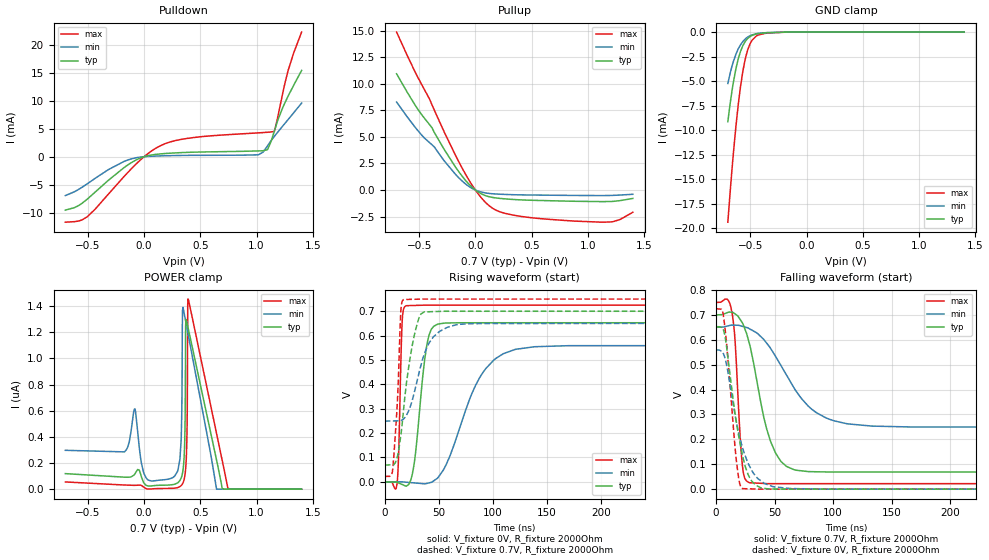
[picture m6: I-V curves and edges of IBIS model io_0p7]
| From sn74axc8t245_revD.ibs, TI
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|   io_0p7 Model
[Model]   io_0p7
Model_type   I/O
Polarity   Non-Inverting
Enable   Active-High
Vinl = 0.21
Vinh = 0.49
Vmeas = 0.35
Vref = 0
Cref = 2pF
Rref = 100000
|   typ   min   max
C_comp   1.54049E-12   1.37923E-12   1.78504E-12
[Model spec]
|subparameter
Vinl   0.21   0.195   0.225
Vinh   0.49   0.455   0.525
| Where Nom  PVT is Nominal Process, 0.7V, 27C
|   Fast PVT is Strong Process,  0.75V, -40C
|   Slow PVT is Weak Process,   0.65, 130C
[Voltage Range]   0.7   0.65   0.75
|Junction Temperature
[Temperature Range]   27   130   -40
[Pullup Reference]   0.7   0.65   0.75
[Pulldown Reference]   0   0   0
[Power Clamp Reference]   0.7   0.65   0.75
[GND Clamp Reference]   0   0   0
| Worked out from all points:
|   slope of the pulldown table from 0 to 0.105 V, typ, clamps not added: 251 ohm
|   slope of the pullup table from 0 to 0.105 V, typ, clamps not added: 180 ohm
|   GND clamp passes 1 mA (typ) near -0.55 V on its own axis
|   falling waveform, V_fixture 0.7V, R_fixture 2000Ohm: 20-80 % time 17.3ns typ, 33.8ns min, 5.11ns max; typ from 0.7 V to 0.069 V
|   rising waveform, V_fixture 0V, R_fixture 2000Ohm: 20-80 % time 8.82ns typ, 29.9ns min, 2.41ns max; typ from 0 V to 0.653 V
|   rising waveform, V_fixture 0.7V, R_fixture 2000Ohm: 20-80 % time 11ns typ, 16ns min, 4.59ns max; typ from 0.069 V to 0.7 V
|   falling waveform, V_fixture 0V, R_fixture 2000Ohm: 20-80 % time 12.5ns typ, 15.7ns min, 7.58ns max; typ from 0.653 V to 0 V
[Pulldown]
|   Voltage   I(typ)   I(min)   I(max)
-700mV    -9.53mA    -6.936mA   -11.68mA
-504.7mV  -7.56mA    -4.826mA   -10.71mA
-116.2mV  -1.094mA   -401.5uA   -2.212mA
-700uV    -4.135uA   -1.175uA   -12.02uA
156.8mV   524.2uA    153.9uA    2.074mA
444.5mV   814.4uA    247.4uA    3.433mA
1.016V    1.034mA    340.2uA    4.259mA
1.058V    1.067mA    839.6uA    4.313mA
1.098V    1.317mA    1.959mA    4.368mA
1.156V    4.475mA    3.596mA    4.506mA
1.278V    10.74mA    6.591mA    15.25mA
1.4V      15.4mA     9.579mA    22.24mA
[GND Clamp]
|   Voltage   I(typ)   I(min)   I(max)
-700mV    -9.134mA   -5.242mA   -19.38mA
-664.3mV  -6.083mA   -3.529mA   -14.17mA
-630.7mV  -3.882mA   -2.333mA   -9.91mA
-605.5mV  -2.655mA   -1.67mA    -7.215mA
-567.7mV  -1.415mA   -980.1uA   -4.082mA
-544.6mV  -944.1uA   -698.3uA   -2.722mA
-521.5mV  -629.7uA   -495uA     -1.75mA
-483.7mV  -335.9uA   -282.4uA   -814.3uA
-445.9mV  -193.6uA   -164.6uA   -387.5uA
-351.4mV  -64.76uA   -49.97uA   -92.43uA
-175mV    -4.252uA   -4.028uA   -4.183uA
1.4V      0A         0A         0A
[Pullup]
|   Voltage   I(typ)   I(min)   I(max)
-700mV    10.94mA    8.279mA    14.86mA
-511mV    7.597mA    5.59mA     10.6mA
-385mV    5.85mA     4.251mA    8.008mA
-275.8mV  3.798mA    2.733mA    5.441mA
-116.2mV  1.282mA    830.6uA    2.039mA
-700uV    5.462uA    3.045uA    10.64uA
129.5mV   -653.1uA   -334uA     -1.541mA
213.5mV   -787.5uA   -396.1uA   -2.037mA
360.5mV   -908.5uA   -451.5uA   -2.409mA
881.3mV   -1.064mA   -514.5uA   -2.93mA
1.222V    -1.075mA   -509.2uA   -2.989mA
1.4V      -796uA     -406uA     -2.097mA
[POWER Clamp]
|   Voltage   I(typ)   I(min)   I(max)
-700mV    118.8nA    297.2nA    55.28nA
-82.6mV   116.1nA    614.3nA    29.33nA
18.2mV    29.94nA    86.4nA     4.018nA
255.5mV   34.86nA    88.97nA    6.633nA
318.5mV   66.18nA    231.3nA    19.67nA
337.4mV   106.9nA    801.1nA    35.29nA
341.6mV   123.5nA    1.369uA    41.03nA
360.5mV   347.9nA    1.325uA    93.15nA
379.4mV   1.28uA     1.24uA     350.7nA
389.9mV   1.239uA    1.192uA    1.454uA
744.8mV   0A         0A         6.021nA
1.4V      0A         0A         0A
[Ramp]
R_load = 2000
|   typ   min   max
dV/dt_r   0.391697/8.77565e-09   0.335547/2.98927e-08   0.434999/2.39639e-09
dV/dt_f   0.378832/1.72731e-08   0.240634/3.38318e-08   0.436699/5.08929e-09
[Falling Waveform]
V_fixture = 0.7V
V_fixture_min = 0.65V
V_fixture_max = 0.75V
R_fixture = 2000Ohm
C_fixture = 0F
|   Time   V(typ)   V(min)   V(max)
0s        700mV      650mV      750mV
13.57ns   710.5mV    659mV      711mV
16.42ns   703.2mV    658.6mV    584.9mV
22.45ns   668.6mV    654.1mV    98.27mV
28.31ns   587.6mV    644.9mV    26.3mV
46.67ns   191mV      564.7mV    22.2mV
67.52ns   77.03mV    399.7mV    22.2mV
93.66ns   69.19mV    286.8mV    22.2mV
133.2ns   68.71mV    253.3mV    22.19mV
500ns     68.61mV    248.9mV    22.17mV
[Rising Waveform]
V_fixture = 0V
V_fixture_min = 0V
V_fixture_max = 0V
R_fixture = 2000Ohm
C_fixture = 0F
|   Time   V(typ)   V(min)   V(max)
0s        923.3nV    12.36uV    39.3nV
11.32ns   -1.698mV   -323.5uV   -9.278mV
16.05ns   -11mV      -463.7uV   653.2mV
19.76ns   -18.13mV   -1.707mV   722.7mV
27.05ns   70.28mV    -4.537mV   723.7mV
39.15ns   566mV      -6.545mV   725mV
48.98ns   647.1mV    15.97mV    725mV
87.49ns   652.8mV    425mV      725mV
120.3ns   652.8mV    542.7mV    725mV
500ns     652.8mV    559.3mV    725mV
[Rising Waveform]
V_fixture = 0.7V
V_fixture_min = 0.65V
V_fixture_max = 0.75V
R_fixture = 2000Ohm
C_fixture = 0F
|   Time   V(typ)   V(min)   V(max)
0s        68.61mV    248.9mV    22.17mV
7.377ns   69.87mV    249.7mV    52.86mV
11.84ns   106.3mV    250.2mV    345.4mV
14.84ns   190mV      251mV      699mV
17.61ns   305.8mV    259mV      748.1mV
27.36ns   602mV      367.3mV    749.1mV
36.62ns   697.3mV    524.4mV    750mV
50.9ns    699.3mV    617.7mV    750mV
78.59ns   700mV      648.9mV    750mV
500ns     700mV      650mV      750mV
[Falling Waveform]
|Gnd
V_fixture = 0V
V_fixture_min = 0V
V_fixture_max = 0V
R_fixture = 2000Ohm
C_fixture = 0F
|   Time   V(typ)   V(min)   V(max)
0s        652.8mV    559.3mV    725mV
6.315ns   639.8mV    543.9mV    697.6mV
9.387ns   557.7mV    489.8mV    566.2mV
17.34ns   269.7mV    270.9mV    114.8mV
20.19ns   192.1mV    209.1mV    22.56mV
22.68ns   134.3mV    165.5mV    2.15mV
27.67ns   55.65mV    101.2mV    1.438mV
34.21ns   15.08mV    50.52mV    576.2uV
63.11ns   71.4uV     2.653mV    22.92uV
500ns     923.6nV    12.38uV    138.7nV
